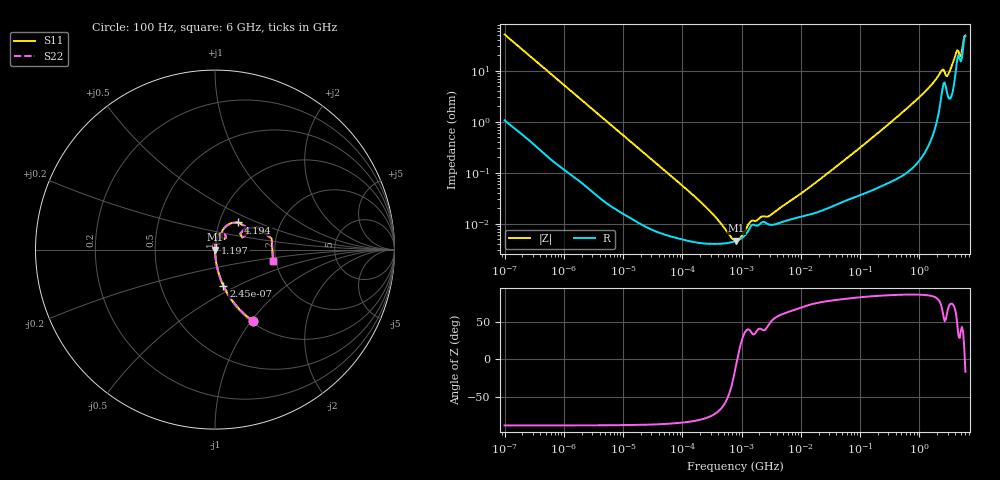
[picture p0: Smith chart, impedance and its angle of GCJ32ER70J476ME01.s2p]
!Murata Part Number: GCJ32ER70J476ME01
!These Parameters are Measured in Series Mode Connection
!Data Generated on Mar 13, 2026
!  o--ll--o
!Port1  Port2
!  o------o
!Operation Temp=25[degC], DC Bias Voltage=0[V]
!Freq. Start=100[Hz] Stop=6[GHz] 401[Steps]
# Hz S RI R 50
!Freq.(Hz) S11(Real) S11(Imag) S21(Real) S21(Imag) S12(Real) S12(Imag) S22(Real) S22(Imag)
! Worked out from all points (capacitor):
!   401 points, 100 Hz to 6 GHz, reference 50 ohm
!   read as one part in series: C = 31 uF near 109 Hz
!   lowest |Z| = 4.63 mohm at 810.1 kHz (marker M1)
!   series resonance near 847.8 kHz, so ESL is about 1.1 nH
!   S11 on the Smith chart (normalised r, x): 100 Hz: 1.02, -1.02; 245 Hz: 1.01, -0.42; 1.197 GHz: 1.00, +0.07; 4.194 GHz: 1.23, +0.39; 6 GHz: 1.93, -0.28
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100  0.2125 -0.3988  0.7875 0.3988  0.7875 0.3988  0.2125 -0.3988
245  0.0468 -0.2008  0.9532 0.2008  0.9532 0.2008  0.0468 -0.2008
627  0.00865 -0.0828  0.9913 0.0828  0.9913 0.0828  0.00865 -0.0828
2008  0.00133 -0.0265  0.9987 0.0265  0.9987 0.0265  0.00133 -0.0265
40335  6.87e-05 -0.00137  0.9999 0.00137  0.9999 0.00137  6.87e-05 -0.00137
193316  4.22e-05 -0.000279  1 0.000279  1 0.000279  4.22e-05 -0.000279
432798  4.04e-05 -9.84e-05  1 9.84e-05  1 9.84e-05  4.04e-05 -9.84e-05
495019  4.09e-05 -7.69e-05  1 7.69e-05  1 7.69e-05  4.09e-05 -7.69e-05
774597  4.51e-05 -1.25e-05  1 1.25e-05  1 1.25e-05  4.51e-05 -1.25e-05
810067  4.59e-05 -6.3e-06  1 6.3e-06  1 6.3e-06  4.59e-05 -6.3e-06
1212075  6.44e-05 5.24e-05  0.9999 -5.24e-05  0.9999 -5.24e-05  6.44e-05 5.24e-05
2169299  0.000105 8.92e-05  0.9999 -8.92e-05  0.9999 -8.92e-05  0.000105 8.92e-05
2967816  9.58e-05 0.000107  0.9999 -0.000107  0.9999 -0.000107  9.58e-05 0.000107
1.555665e7  0.000156 0.000545  0.9998 -0.000545  0.9998 -0.000545  0.000156 0.000545
3.124326e8  0.000725 0.00918  0.9993 -0.00918  0.9993 -0.00918  0.000725 0.00918
1.197065e9  0.00366 0.0366  0.9963 -0.0366  0.9963 -0.0366  0.00366 0.0366
2.34314e9  0.0369 0.0872  0.9631 -0.0872  0.9631 -0.0872  0.0369 0.0872
3.065283e9  0.0353 0.0725  0.9647 -0.0725  0.9647 -0.0725  0.0353 0.0725
3.666503e9  0.0532 0.1222  0.9468 -0.1222  0.9468 -0.1222  0.0532 0.1222
4.193612e9  0.1289 0.1512  0.8711 -0.1512  0.8711 -0.1512  0.1289 0.1512
5.016141e9  0.1406 0.0888  0.8594 -0.0888  0.8594 -0.0888  0.1406 0.0888
6e9  0.3234 -0.0645  0.6766 0.0645  0.6766 0.0645  0.3234 -0.0645
